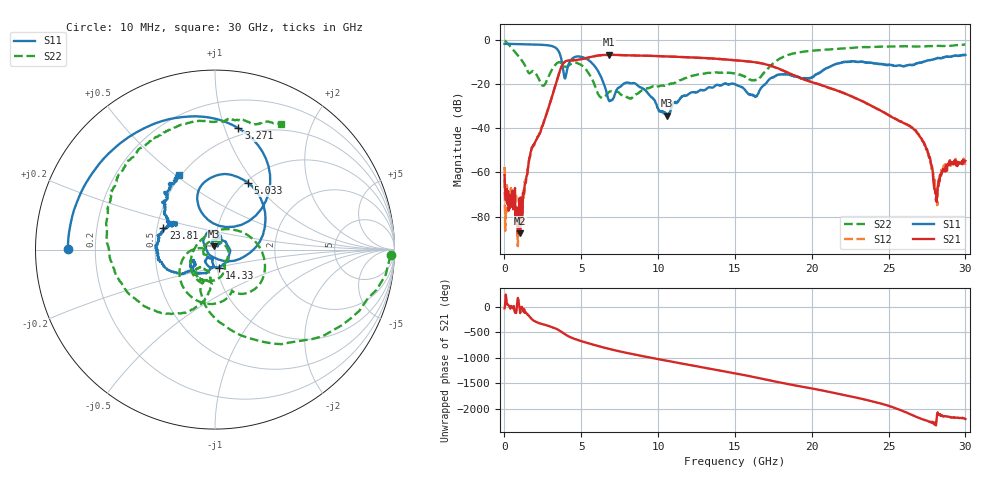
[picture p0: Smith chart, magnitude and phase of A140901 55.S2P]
!  2-Port S-parameters saved by WinCal
! VAR MeasName=S-Parameters (CALIBRATED_DATA) read from VNA (N5244A)
! VAR MeasDate=11/3/2014 9:36:13 AM
! VAR NAME=A140901 55
! VAR FILENAME=A140901 55.S2P
! VAR DATE=11/3/2014 9:36:13 AM
! VAR PHYS_PORTS=1,2
# Hz S RI R 50
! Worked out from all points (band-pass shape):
!   801 points, 10 MHz to 30 GHz, reference 50 ohm
!   highest |S21| = -6.66 dB at 6.795 GHz (marker M1); lowest = -87.6 dB at 1.022 GHz (marker M2)
!   |S21| within 3 dB of the highest: 3.966 GHz to 15.8 GHz (11.84 GHz wide, 120 % of centre)
!   lowest |S11| = -34.2 dB at 10.58 GHz (marker M3), VSWR 1.04, Z = 49.3 + j1.78 ohm
!   |S11| at or under -10 dB: 3.743 GHz to 4.237 GHz (494.7 MHz wide, 12.4 % of centre); 5.63 GHz to 22.07 GHz (16.44 GHz wide, 119 % of centre); 23.42 GHz to 27.23 GHz (3.811 GHz wide, 15 % of centre)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
!   |S22| runs from -26.6 to -0.2 dB; largest |S21 - S12| = 0.0029
!   S11 on the Smith chart (normalised r, x): 10 MHz: 0.10, +0.00; 3.271 GHz: 0.43, +1.11; 5.033 GHz: 1.03, +0.92; 14.33 GHz: 1.03, -0.21; 23.81 GHz: 0.54, +0.14; 30 GHz: 0.49, +0.52
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1e7  -0.8185 0.00342  0.00075 -0.000423  6.97e-06 0.00133  0.9782 -0.0322
1.022162e9  -0.743 0.3248  -2.27e-05 -3.49e-05  0.000109 -2.72e-05  0.00911 -0.3888
1.734425e9  -0.601 0.5266  -0.00217 0.00223  -0.00219 0.00223  -0.0478 -0.1816
2.521662e9  -0.3314 0.7038  0.0123 0.00368  0.0122 0.00366  -0.0565 0.0728
3.271412e9  0.1305 0.6764  0.0454 -0.0705  0.0455 -0.0703  0.2641 -0.0183
3.946188e9  0.0223 0.1324  -0.3256 -0.00842  -0.3251 -0.00864  0.0954 -0.229
5.033325e9  0.1849 0.3709  0.2606 0.2627  0.26 0.2627  -0.1859 -0.1916
6.795238e9  -0.0103 -0.0421  -0.1038 -0.4527  -0.103 -0.4526  -0.0599 -0.0277
8.1073e9  -0.0199 0.1052  -0.4405 0.0911  -0.4405 0.0909  0.00501 0.0477
1.001916e10  0.0152 0.0221  0.2496 0.3551  0.2491 0.3544  0.0574 -0.067
1.058148e10  -0.00714 0.0181  0.3926 0.1678  0.3926 0.1674  0.0524 -0.079
1.249334e10  0.0373 0.0531  0.0528 -0.3947  0.052 -0.3945  0.0158 -0.1618
1.433022e10  0.0248 -0.1007  -0.3624 0.0291  -0.3642 0.0276  -0.0839 -0.1621
1.5005e10  -0.0368 -0.0918  -0.2565 0.2352  -0.2568 0.2348  -0.1063 -0.1384
1.702932e10  -0.0183 -0.1032  0.2708 0.0712  0.2704 0.0725  -0.0211 -0.2047
2.002832e10  -0.1144 -0.0851  -0.104 -0.0376  -0.104 -0.0392  -0.56 -0.116
2.381456e10  -0.2873 0.1206  0.0249 -0.0222  0.025 -0.0223  -0.4352 0.5464
2.501416e10  -0.2245 0.1502  -0.0151 -0.0128  -0.0151 -0.013  -0.2717 0.6602
2.715095e10  -0.2643 0.1705  0.00458 -0.00339  0.00471 -0.00349  0.0176 0.713
2.808814e10  -0.2842 0.2591  -0.000336 -9.96e-05  -0.000184 0.000138  0.1483 0.7267
2.883789e10  -0.2788 0.3116  0.0015 0.000233  0.0015 -1.29e-05  0.2203 0.6993
3e10  -0.1986 0.4157  0.00145 -0.00112  0.00126 -0.000811  0.3672 0.7016
